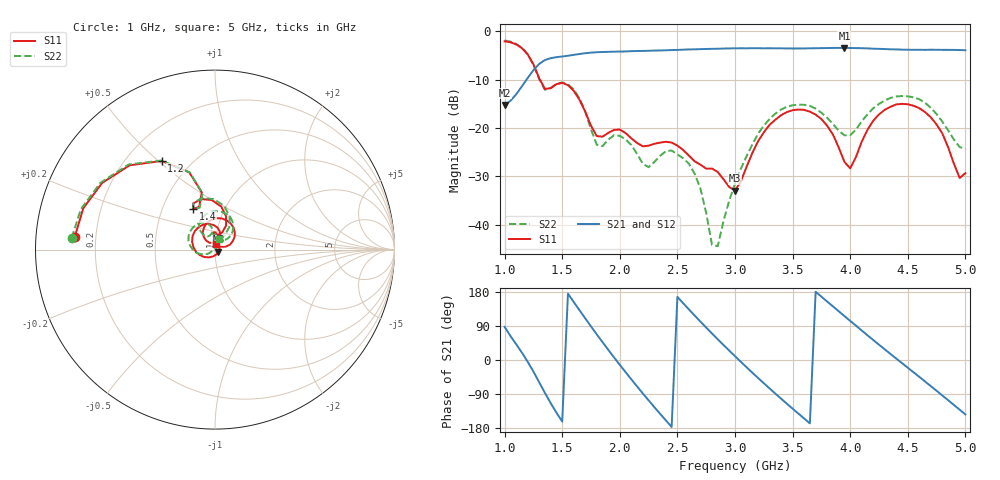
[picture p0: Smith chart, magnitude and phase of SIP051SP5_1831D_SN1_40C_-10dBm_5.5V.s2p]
# GHz  S  dB  R  50
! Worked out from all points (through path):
!   81 points, 1 GHz to 5 GHz, reference 50 ohm
!   highest |S21| = -3.45 dB at 3.95 GHz (marker M1); lowest = -15.3 dB at 1 GHz (marker M2)
!   lowest |S11| = -32.9 dB at 3 GHz (marker M3), VSWR 1.05, Z = 51.9 - j1.23 ohm
!   |S11| at or under -10 dB: 1.307 GHz to end of sweep
!   |S22| runs from -44.4 to -1.9 dB; largest |S21 - S12| = 0.0027
!   S11 on the Smith chart (normalised r, x): 1 GHz: 0.12, +0.04; 1.2 GHz: 0.35, +0.51; 1.4 GHz: 0.71, +0.35; 5 GHz: 1.01, +0.07
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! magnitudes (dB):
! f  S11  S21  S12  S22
! 1 GHz  -2.1  -15.3  -15.3  -1.9
! 1.2 GHz  -4.8  -9.7  -9.7  -4.7
! 1.4 GHz  -11.8  -5.6  -5.6  -11.8
! 1.55 GHz  -11.2  -5.1  -5.1  -11.0
! 1.7 GHz  -16.6  -4.6  -4.6  -16.6
! 1.8 GHz  -21.7  -4.4  -4.4  -23.5
! 2 GHz  -20.3  -4.2  -4.2  -21.6
! 2.25 GHz  -23.7  -4.0  -4.0  -28.1
! 2.35 GHz  -23.0  -4.0  -4.0  -25.7
! 2.6 GHz  -25.7  -3.8  -3.8  -27.4
! 2.7 GHz  -27.6  -3.7  -3.7  -32.5
! 2.8 GHz  -28.4  -3.6  -3.6  -44.1
! 2.85 GHz  -29.1  -3.6  -3.6  -44.4
! 3 GHz  -32.9  -3.5  -3.5  -31.5
! 3.3 GHz  -19.3  -3.5  -3.5  -18.2
! 3.7 GHz  -17.2  -3.5  -3.5  -16.0
! 3.95 GHz  -27.0  -3.5  -3.5  -21.5
! 4 GHz  -28.3  -3.5  -3.5  -21.5
! 4.35 GHz  -15.6  -3.7  -3.7  -13.8
! 4.65 GHz  -16.7  -3.9  -3.8  -14.8
! 4.95 GHz  -30.3  -3.9  -3.9  -23.9
! 5 GHz  -29.3  -3.9  -3.9  -24.3
